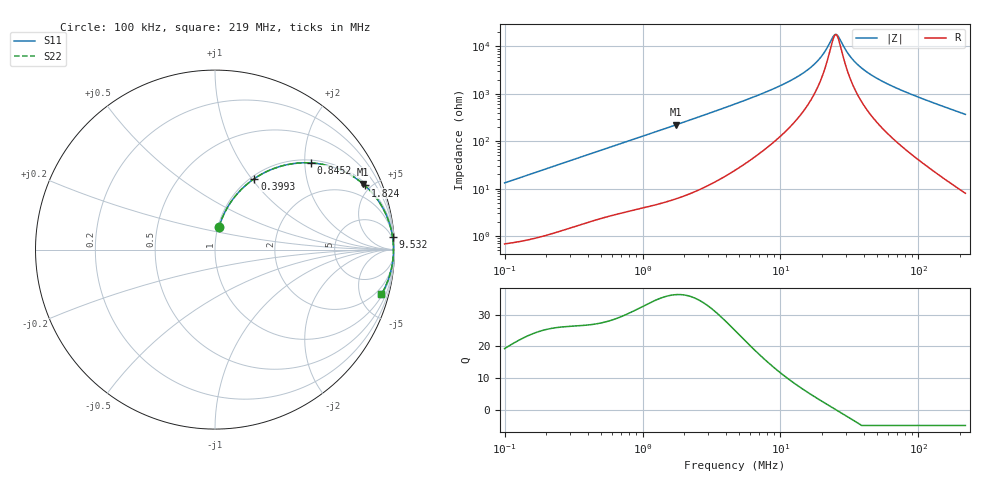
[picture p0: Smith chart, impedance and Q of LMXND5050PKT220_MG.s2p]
! LMXND5050PKT220_MG  S-PARAMETER MODEL  ( General Type )
! Model Generated by TAIYO YUDEN Corporation (https://www.yuden.co.jp/en/)
! Version 1.0
! TAIYO YUDEN Control No. 191023NI43SB-FBB
! Copyright(c) 2019 TAIYO YUDEN CO.,LTD. All Rights Reserved.
! Product Description (link to TY-COMPAS)
! https://ds.yuden.co.jp/TYCOMPAS/or/detail?pn=LMXND5050PKT220MMG&u=M
! Products Name : Inductors
! Characteristics :
!  Inductance : 22 uH , SRF(min) : 16 MHz , DC Resistance(max) : 0.54 Ohm
!  Rated Current : Saturation :900 mA , Temp Rise : 550 mA (40 degC)
!  Case Size : 4.9 x 4.9 / 0.193 x 0.193 [mm/inch] , Thickness : 1.4 / 0.055 [mm/inch]
!  (Conditions: Temperature = 25 degC , DC Bias Current/Voltage = 0A / 0V)
! External Node Assignments :
!  1  o---GGG---o  2
! GND o---------o GND
! Frequency Range : 0.1MHz  -  218.972167MHz  [ 402 STEP ]
# MHz S RI R 50
! Freq[MHz].  S11 Real  S11 Imag  S21 Real  S21 Imag  S12 Real  S12 Imag  S22 Real  S22 Imag
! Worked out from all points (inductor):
!   401 points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, 100 kHz to 219 MHz, reference 50 ohm
!   read as one part in series: L = 20.9 uH near 103.9 kHz
!   highest Q = 36.3 at 1.755 MHz (marker M1), where L = 20.2 uH
!   self-resonance near 24.93 MHz
!   S11 on the Smith chart (normalised r, x): 100 kHz: 1.01, +0.26; 399.3 kHz: 1.04, +1.03; 845.2 kHz: 1.07, +2.15; 1.824 MHz: 1.13, +4.62; 9.532 MHz: 3, +28; 219 MHz: 1.16, -7.36
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0.1  0.0235 0.1279  0.9765 -0.1279  0.9765 -0.1279  0.0235 0.1279
0.207652  0.0774 0.2483  0.9226 -0.2483  0.9226 -0.2483  0.0774 0.2483
0.362673  0.1903 0.3742  0.8097 -0.3742  0.8097 -0.3742  0.1903 0.3742
0.399273  0.2194 0.3956  0.7806 -0.3956  0.7806 -0.3956  0.2194 0.3956
0.845197  0.5356 0.4829  0.4644 -0.4829  0.4644 -0.4829  0.5356 0.4829
1.315317  0.7296 0.4301  0.2704 -0.4301  0.2704 -0.4301  0.7296 0.4301
1.755072  0.8251 0.3664  0.1749 -0.3664  0.1749 -0.3664  0.8251 0.3664
1.823882  0.8356 0.3571  0.1644 -0.3571  0.1644 -0.3571  0.8356 0.3571
4.770297  0.9688 0.1547  0.0312 -0.1547  0.0312 -0.1547  0.9688 0.1547
9.531921  0.9892 0.0703  0.0108 -0.0703  0.0108 -0.0703  0.9892 0.0703
13.21743  0.9925 0.043  0.00751 -0.043  0.00751 -0.043  0.9925 0.043
16.97108  0.9938 0.0253  0.00624 -0.0253  0.00624 -0.0253  0.9938 0.0253
20.17755  0.9942 0.0139  0.00577 -0.0139  0.00577 -0.0139  0.9942 0.0139
23.98983  0.9944 0.00299  0.00557 -0.00299  0.00557 -0.00299  0.9944 0.00299
25.41441  0.9944 -0.000618  0.00556 0.000618  0.00556 0.000618  0.9944 -0.000618
26.41082  0.9944 -0.00302  0.00556 0.00302  0.00556 0.00302  0.9944 -0.00302
31.4008  0.9943 -0.014  0.00574 0.014  0.00574 0.014  0.9943 -0.014
36.62254  0.9939 -0.024  0.00612 0.024  0.00612 0.024  0.9939 -0.024
45.24902  0.9929 -0.0388  0.00706 0.0388  0.00706 0.0388  0.9929 -0.0388
61.54953  0.9904 -0.0634  0.00961 0.0634  0.00961 0.0634  0.9904 -0.0634
107.4986  0.9786 -0.1242  0.0214 0.1242  0.0214 0.1242  0.9786 -0.1242
218.9722  0.9266 -0.2501  0.0734 0.2501  0.0734 0.2501  0.9266 -0.2501
